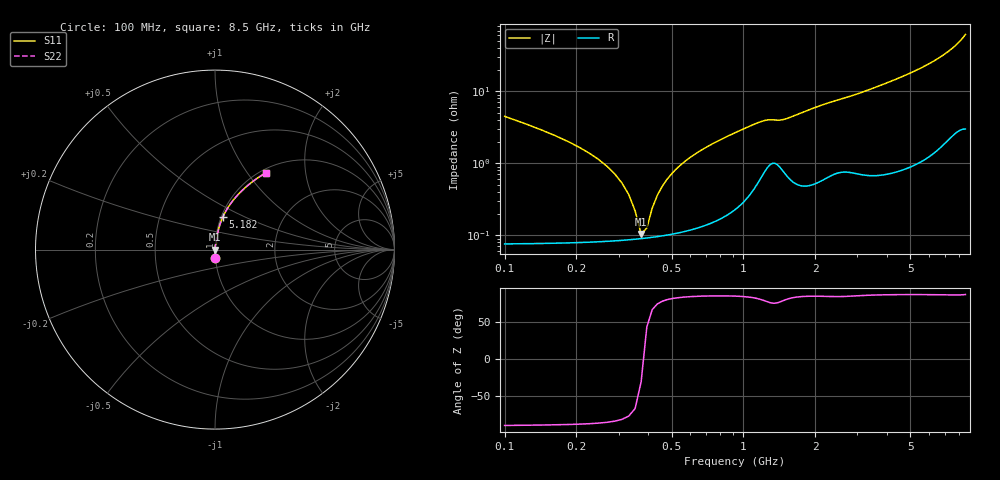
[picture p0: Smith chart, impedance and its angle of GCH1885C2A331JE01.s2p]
!Murata Part Number: GCH1885C2A331JE01
!These Parameters are Measured in Series Mode Connection
!Data Generated on Jun 19, 2026
!  o--ll--o
!Port1  Port2
!  o------o
!Operation Temp=25[degC], DC Bias Voltage=0[V]
!Freq. Start=100[MHz] Stop=9[GHz] 401[Steps]
# Hz S RI R 50
!Freq.(Hz) S11(Real) S11(Imag) S21(Real) S21(Imag) S12(Real) S12(Imag) S22(Real) S22(Imag)
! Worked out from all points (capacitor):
!   401 points, 100 MHz to 8.5 GHz, reference 50 ohm
!   read as one part in series: C = 330 pF near 142 MHz
!   lowest |Z| = 104 mohm at 373 MHz (marker M1)
!   series resonance near 380.9 MHz, so ESL is about 530 pH
!   S11 on the Smith chart (normalised r, x): 100 MHz: 1.00, -0.09; 5.182 GHz: 1.02, +0.38; 8.5 GHz: 1.06, +1.23
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1e8  0.00277 -0.0448  0.9972 0.0448  0.9972 0.0448  0.00277 -0.0448
1.42e8  0.00162 -0.0292  0.9984 0.0292  0.9984 0.0292  0.00162 -0.0292
2.68e8  0.000906 -0.00909  0.9991 0.00909  0.9991 0.00909  0.000906 -0.00909
3.1e8  0.000877 -0.00525  0.9991 0.00525  0.9991 0.00525  0.000877 -0.00525
3.52e8  0.000885 -0.002  0.9991 0.002  0.9991 0.002  0.000885 -0.002
3.73e8  0.000898 -0.000523  0.9991 0.000523  0.9991 0.000523  0.000898 -0.000523
3.94e8  0.000917 0.00087  0.9991 -0.00087  0.9991 -0.00087  0.000917 0.00087
4.15e8  0.000941 0.00219  0.9991 -0.00219  0.9991 -0.00219  0.000941 0.00219
4.57e8  0.001 0.00468  0.999 -0.00468  0.999 -0.00468  0.001 0.00468
5.2e8  0.00112 0.00809  0.9989 -0.00809  0.9989 -0.00809  0.00112 0.00809
6.04e8  0.00134 0.0122  0.9987 -0.0122  0.9987 -0.0122  0.00134 0.0122
7.09e8  0.0017 0.0171  0.9983 -0.0171  0.9983 -0.0171  0.0017 0.0171
8.98e8  0.00276 0.0253  0.9972 -0.0253  0.9972 -0.0253  0.00276 0.0253
1.15e9  0.0066 0.0358  0.9934 -0.0358  0.9934 -0.0358  0.0066 0.0358
1.507e9  0.0085 0.0403  0.9915 -0.0403  0.9915 -0.0403  0.0085 0.0403
2.116e9  0.00962 0.0627  0.9904 -0.0627  0.9904 -0.0627  0.00962 0.0627
2.914e9  0.0149 0.087  0.9851 -0.087  0.9851 -0.087  0.0149 0.087
4.3e9  0.0275 0.1397  0.9725 -0.1397  0.9725 -0.1397  0.0275 0.1397
5.182e9  0.043 0.1797  0.957 -0.1797  0.957 -0.1797  0.043 0.1797
5.707e9  0.0564 0.2071  0.9436 -0.2071  0.9436 -0.2071  0.0564 0.2071
7.114e9  0.1211 0.2984  0.8789 -0.2984  0.8789 -0.2984  0.1211 0.2984
8.5e9  0.2848 0.4277  0.7152 -0.4277  0.7152 -0.4277  0.2848 0.4277
